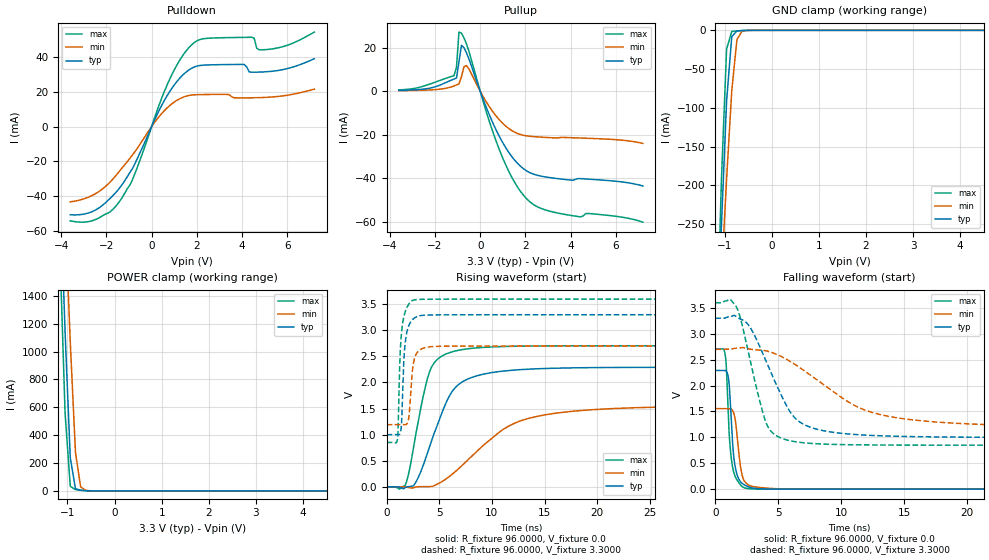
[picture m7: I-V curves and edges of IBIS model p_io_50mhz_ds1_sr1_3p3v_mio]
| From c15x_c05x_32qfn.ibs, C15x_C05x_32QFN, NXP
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[Model] p_io_50mhz_ds1_sr1_3p3v_mio
|   Model p_io_50mhz_ds1_sr1_3p3v_mio
| This model was characterised for following simulation conditions:
| External (pad) voltage:
|   - Typ: 3.3V,   - Min: 2.7V,   - Max: 3.6V
| Library cells for typ/min/max conditions are connected as defined below:
|  pad - External Pad
|  ipp_do_lv - Core Input
|  ipp_obe_lv - Output Buffer Enable
|  IOGC - NC
|  REFH3V3 - REFH3V3
|  REFL3V3 - REFL3V3
|  ZI - NC
|  abut_ncal_vddio[1] - vddio
|  abut_ncal_vddio[2] - vddio
|  abut_ncal_vddio[3] - vssio
|  abut_ncal_vddio[4] - vddio
|  abut_ncal_vddio[5] - vddio
|  abut_ncal_vddio[6] - vssio
|  abut_pcal_vddio[1] - vssio
|  abut_pcal_vddio[2] - vssio
|  abut_pcal_vddio[3] - vddio
|  abut_pcal_vddio[4] - vssio
|  abut_pcal_vddio[5] - vssio
|  abut_pcal_vddio[6] - vddio
|  ipp_do_1p8v - ipp_do_1p8v
|  ipp_dse_lv - vdd_lv
|  ipp_eftd_lv - NC
|  ipp_ina_mux_vddio - NC
|  ipp_ina_mux_vddio[0] - NC
|  ipp_ina_mux_vddio[1] - NC
|  ipp_ina_r0_vddio - NC
|  ipp_ina_r0a_vddio - NC
|  ipp_ina_r0b_vddio - NC
|  ipp_ina_r0c_vddio - NC
|  ipp_ina_r0d_vddio - NC
|  ipp_ina_r0e_vddio - NC
|  ipp_ina_r0f_vddio - NC
|  ipp_ina_r300_vddio - NC
|  ipp_ina_r300a_vddio - NC
|  ipp_ina_r300b_vddio - NC
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Model_type I/O
Polarity   Non-Inverting
Enable   Active-High
Vinl =   0.9900V
Vinh =   2.3100V
Vmeas =  1.6500V
Cref =   30.0000pF
Rref =   1.0000M
Vref =   3.3000V
C_comp   1.4363pF   1.3758pF   1.5227pF
|C_comp_pullup   0.7209pF   0.7531pF   0.6989pF
|C_comp_pulldown   0.6266pF   0.6811pF   0.5874pF
[Model Spec]
| variable   typ   min   max
Vinh   2.3100V   1.8900V   2.5200V
Vinl   0.9900V   0.8100V   1.0800V
[Temperature Range]   25.0000   0.1250k   -40.0000
[Voltage Range]   3.3000V   2.7000V   3.6000V
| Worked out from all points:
|   slope of the pulldown table from 0 to 0.495 V, typ, clamps not added: 36.8 ohm
|   slope of the pullup table from 0 to 0.495 V, typ, clamps not added: 37.8 ohm
|   GND clamp passes 1 mA (typ) near -0.74 V on its own axis
|   POWER clamp passes 1 mA (typ) near -0.54 V on its own axis
|   rising waveform, R_fixture 96.0000, V_fixture 0.0: 20-80 % time 2.69ns typ, 5.82ns min, 1.63ns max; typ from 0 V to 2.29 V
|   rising waveform, R_fixture 96.0000, V_fixture 3.3000: 20-80 % time 349ps typ, 388ps min, 335ps max; typ from 0.998 V to 3.3 V
|   falling waveform, R_fixture 96.0000, V_fixture 0.0: 20-80 % time 404ps typ, 456ps min, 385ps max; typ from 2.29 V to 0 V
|   falling waveform, R_fixture 96.0000, V_fixture 3.3000: 20-80 % time 2.66ns typ, 5.9ns min, 1.62ns max; typ from 3.3 V to 0.998 V
[Pulldown]
|Voltage   I(typ)   I(min)   I(max)
-3.6V     -50.71mA   -43.27mA   -54.18mA
-2.5V     -48.1mA    -38.69mA   -53.56mA
-1.4V     -35.02mA   -25.26mA   -42.7mA
-850mV    -24.18mA   -16.32mA   -30.7mA
800mV     20.23mA    12.14mA    27.32mA
1.9V      34.45mA    18.38mA    48.57mA
4.1V      35.83mA    16.63mA    51.44mA
4.43V     31.42mA    16.66mA    51.52mA
4.54V     31.41mA    16.69mA    50.94mA
4.65V     31.42mA    16.71mA    45.28mA
5.09V     31.67mA    16.92mA    44.44mA
7.2V      39.12mA    21.58mA    54.49mA
[Pullup]
|Voltage   I(typ)   I(min)   I(max)
-3.6V     390.2uA    234.7uA    600.5uA
-1.16V    5.607mA    2.418mA    7.152mA
-1.05V    6.059mA    2.87mA     11.01mA
-940mV    13.57mA    3.339mA    27.22mA
-830mV    21.13mA    6.682mA    26.77mA
-720mV    20.02mA    11.25mA    24.57mA
-610mV    17.72mA    11.8mA     21.82mA
820mV     -20.27mA   -12.85mA   -26.19mA
1.48V     -31.2mA    -18.62mA   -41.17mA
2.03V     -36.53mA   -20.52mA   -49.25mA
3.46V     -40.29mA   -21.45mA   -56.15mA
7.2V      -43.65mA   -24.03mA   -60.31mA
[GND_clamp]
|Voltage   I(typ)   I(min)   I(max)
-3.6V     -4.967A    -3.834A    -6.451A
-1.18V    -432.4mA   -454.2mA   -428.7mA
-1.07V    -252.8mA   -319.9mA   -193.4mA
-960mV    -91.54mA   -192mA     -24.27mA
-850mV    -8.013mA   -77.88mA   -1.462mA
-740mV    -731.9uA   -11.92mA   -724.8uA
-630mV    -284.5uA   -927.4uA   -315.1uA
-300mV    -508.9nA   -3.017uA   -108.6nA
7.2V      0A         0A         0A
[POWER_clamp]
|Voltage   I(typ)   I(min)   I(max)
-3.6V     26.34A     23.98A     28.82A
-1.16V    2.208A     2.937A     1.722A
-1.05V    1.14A      1.999A     556.4mA
-940mV    237.9mA    1.069A     33.46mA
-830mV    16.33mA    277.1mA    9.216mA
-720mV    4.663mA    29.2mA     4.86mA
-610mV    1.877mA    3.923mA    1.821mA
7.2V      0A         0A         0A
[Ramp]
| variable   typ   min   max
dV/dt_r  1.3753/2.6891n   0.9330/5.8229n   1.6230/1.6338n
dV/dt_f  1.3812/2.6604n   0.9059/5.8993n   1.6510/1.6183n
R_load = 96.0000
[Rising Waveform]
R_fixture= 96.0000
V_fixture= 0.0
V_fixture_min= 0.0
V_fixture_max= 0.0
|time   V(typ)   V(min)   V(max)
0s        4.193nV    211.1nV    14.22nV
1.819ns   -10.47mV   -3.924mV   56.67mV
2.848ns   115.4mV    -1.641mV   1.09V
3.764ns   579.8mV    3.089mV    1.99V
4.385ns   958.6mV    10.26mV    2.338V
6.141ns   1.803V     226.3mV    2.584V
8.163ns   2.102V     600.8mV    2.657V
13.11ns   2.252V     1.29V      2.698V
22.42ns   2.289V     1.508V     2.705V
127.4ns   2.292V     1.555V     2.705V
[Rising Waveform]
R_fixture= 96.0000
V_fixture= 3.3000
V_fixture_min= 2.7000
V_fixture_max= 3.6000
|time   V(typ)   V(min)   V(max)
0s        998.1mV    1.19V      848.4mV
1.019ns   1V         1.19V      903mV
1.315ns   1.044V     1.19V      2.686V
1.429ns   1.275V     1.192V     2.991V
1.635ns   2.433V     1.191V     3.262V
1.81ns    2.837V     1.192V     3.385V
2.11ns    3.093V     1.332V     3.504V
2.446ns   3.204V     2.231V     3.571V
2.802ns   3.256V     2.542V     3.59V
127.4ns   3.3V       2.7V       3.6V
[Falling Waveform]
R_fixture= 96.0000
V_fixture= 0.0
V_fixture_min= 0.0
V_fixture_max= 0.0
|time   V(typ)   V(min)   V(max)
0s        2.292V     1.555V     2.705V
796.6ps   2.292V     1.555V     2.58V
892.4ps   2.272V     1.555V     2.284V
1.093ns   2.05V      1.557V     1.111V
1.255ns   1.359V     1.548V     625.9mV
1.446ns   673.7mV    1.477V     344.5mV
1.718ns   286.5mV    1.061V     180.2mV
2.106ns   117.7mV    297.5mV    55.14mV
2.705ns   38.92mV    70.4mV     8.843mV
127.4ns   1.805uV    4.006uV    1.24uV
[Falling Waveform]
R_fixture= 96.0000
V_fixture= 3.3000
V_fixture_min= 2.7000
V_fixture_max= 3.6000
|time   V(typ)   V(min)   V(max)
0s        3.3V       2.7V       3.6V
1.151ns   3.332V     2.701V     3.67V
1.743ns   3.318V     2.724V     3.484V
2.805ns   3.107V     2.701V     2.433V
4.243ns   2.345V     2.657V     1.176V
6.005ns   1.467V     2.458V     931.3mV
7.293ns   1.219V     2.245V     889.3mV
12.7ns    1.034V     1.463V     852.7mV
21.64ns   1.002V     1.245V     848.6mV
127.4ns   998.1mV    1.19V      848.4mV
